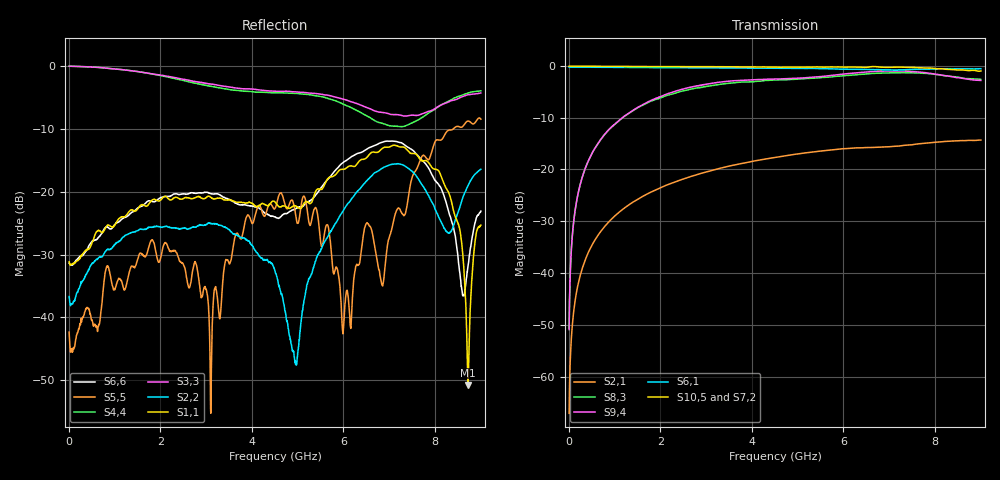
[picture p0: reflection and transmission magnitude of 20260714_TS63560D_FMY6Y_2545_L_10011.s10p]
# GHz S DB R 50
! CMT, SN0916, 25263762, 26.7.0
! Date: 15.07.2026 13:43:35
! Data: Format
! Freq S1.1:dB/Ang S1.2:dB/Ang S1.3:dB/Ang S1.4:dB/Ang S1.5:dB/Ang S1.6:dB/Ang S1.7:dB/Ang S1.8:dB/Ang S1.9:dB/Ang S1.10:dB/Ang
!  S2.1:dB/Ang S2.2:dB/Ang S2.3:dB/Ang S2.4:dB/Ang S2.5:dB/Ang S2.6:dB/Ang S2.7:dB/Ang S2.8:dB/Ang S2.9:dB/Ang S2.10:dB/Ang
!  S3.1:dB/Ang S3.2:dB/Ang S3.3:dB/Ang S3.4:dB/Ang S3.5:dB/Ang S3.6:dB/Ang S3.7:dB/Ang S3.8:dB/Ang S3.9:dB/Ang S3.10:dB/Ang
!  S4.1:dB/Ang S4.2:dB/Ang S4.3:dB/Ang S4.4:dB/Ang S4.5:dB/Ang S4.6:dB/Ang S4.7:dB/Ang S4.8:dB/Ang S4.9:dB/Ang S4.10:dB/Ang
!  S5.1:dB/Ang S5.2:dB/Ang S5.3:dB/Ang S5.4:dB/Ang S5.5:dB/Ang S5.6:dB/Ang S5.7:dB/Ang S5.8:dB/Ang S5.9:dB/Ang S5.10:dB/Ang
!  S6.1:dB/Ang S6.2:dB/Ang S6.3:dB/Ang S6.4:dB/Ang S6.5:dB/Ang S6.6:dB/Ang S6.7:dB/Ang S6.8:dB/Ang S6.9:dB/Ang S6.10:dB/Ang
!  S7.1:dB/Ang S7.2:dB/Ang S7.3:dB/Ang S7.4:dB/Ang S7.5:dB/Ang S7.6:dB/Ang S7.7:dB/Ang S7.8:dB/Ang S7.9:dB/Ang S7.10:dB/Ang
!  S8.1:dB/Ang S8.2:dB/Ang S8.3:dB/Ang S8.4:dB/Ang S8.5:dB/Ang S8.6:dB/Ang S8.7:dB/Ang S8.8:dB/Ang S8.9:dB/Ang S8.10:dB/Ang
!  S9.1:dB/Ang S9.2:dB/Ang S9.3:dB/Ang S9.4:dB/Ang S9.5:dB/Ang S9.6:dB/Ang S9.7:dB/Ang S9.8:dB/Ang S9.9:dB/Ang S9.10:dB/Ang
!  S10.1:dB/Ang S10.2:dB/Ang S10.3:dB/Ang S10.4:dB/Ang S10.5:dB/Ang S10.6:dB/Ang S10.7:dB/Ang S10.8:dB/Ang S10.9:dB/Ang S10.10:dB/Ang
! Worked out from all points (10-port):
!   2001 points, 10 MHz to 9 GHz, reference 50 ohm
!   strongest paths, dB at 10 MHz, 2.257 GHz, 4.505 GHz, 6.753 GHz, 9 GHz:
!     S10,5: -0.1, -0.2, -0.2, -0.2, -1.0
!     S7,2: -0.1, -0.3, -0.4, -0.6, -0.6
!     S6,1: -0.3, -0.4, -0.5, -0.7, -0.6
!     S9,4: -50.9, -5.1, -2.5, -1.0, -2.8
!     S8,3: -50.7, -5.5, -2.7, -1.4, -2.6
!     S2,1: -67.1, -22.6, -17.7, -15.7, -14.3
!   lowest |S11| = -50.8 dB at 8.721 GHz (marker M1), VSWR 1.01, Z = 49.9 + j0.26 ohm
!   |S11| at or under -10 dB: start of sweep to end of sweep
